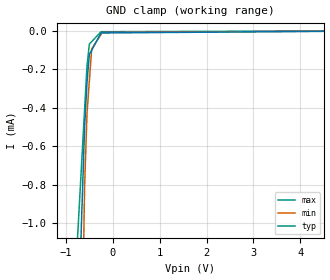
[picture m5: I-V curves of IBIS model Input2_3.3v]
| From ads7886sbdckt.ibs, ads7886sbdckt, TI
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[Model] Input2_3.3v
Model_type Input
Vinl = 400.000mV
Vinh = 4.60000V
C_comp 1.513pF 1.513pF 1.513pF
| variable typ   min   max
[Voltage Range] 3.30000V 3.00000V 3.60000V
[POWER Clamp Reference] 3.30000V 3.00000V 3.60000V
[GND Clamp Reference] 0.00000V 0.00000V 0.00000V
[GND Clamp]
-3.3V     -20.6mA    -39.89mA   -12.35mA
-600mV    -491.1uA   -798uA     -403.4uA
-550mV    -268.7uA   -429.8uA   -182.1uA
-500mV    -122.8uA   -261.3uA   -68.45uA
-450mV    -100.3uA   -92.85uA   -55.58uA
-250mV    -10.46uA   -17.88uA   -4.125uA
-225mV    -10.42uA   -8.51uA    -4.104uA
6.6V      1.321uA    1.798uA    1.647uA
[POWER Clamp]
-3.3V     0A         0A         0A
6.6V      0A         0A         0A
